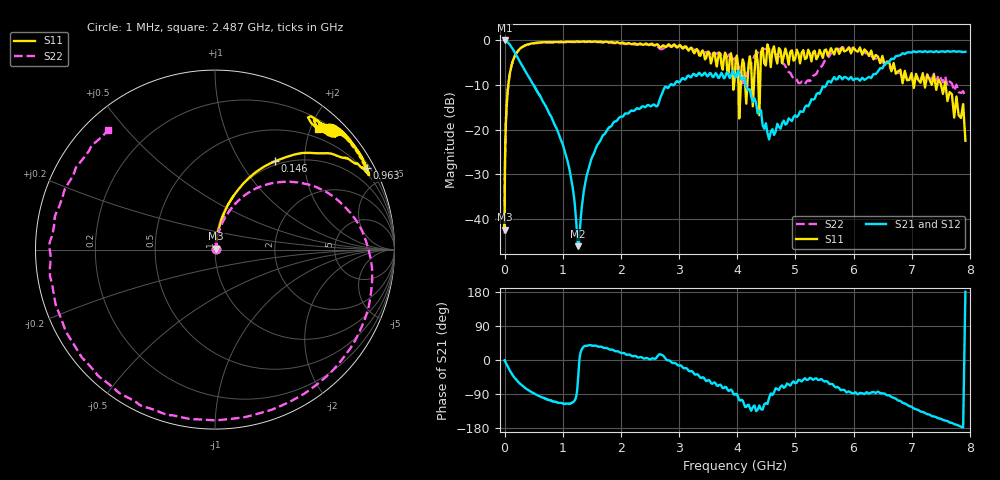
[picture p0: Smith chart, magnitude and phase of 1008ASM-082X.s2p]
!s-Parameter Generated by FASTRON Sdn. Bhd.
!FASTRON P/N : 1008ASM-082X
!Keysight Technologies: E5071C_MY46733604_B.14.02
!Date: Tue Nov 21 11:36:22 2023
!Version  :Rev00  Wed Nov 22 15:52:03 2023
!Data & Calibration Information:
!Freq  S11:SOLT2(ON)  S21:SOLT2(ON)  S12:SOLT2(ON)  S22:SOLT2(ON)
!PortZ  Port1:50+j0  Port2:50+j0
!When reading reference impedance value at option line is always used.
! Remarks : This data is being provided solely for informational purposes.
# Hz S dB R 50
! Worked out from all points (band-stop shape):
!   1599 points, 1 MHz to 7.923 GHz, reference 50 ohm
!   highest |S21| = -0.05 dB at 1.284 MHz (marker M1); lowest = -46.1 dB at 1.264 GHz (marker M2)
!   |S21| within 3 dB of the highest: start of sweep to 188.6 MHz; 6.885 GHz to end of sweep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
!   lowest |S11| = -42.4 dB at 1.31 MHz (marker M3), VSWR 1.02, Z = 50.6 + j0.474 ohm
!   |S11| at or under -10 dB: start of sweep to 64.94 MHz; 4.022 GHz to 4.062 GHz (40.34 MHz wide, 0.998 % of centre); 7.582 GHz to end of sweep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
!   |S22| runs from -43.4 to -0.3 dB; largest |S21 - S12| = 0.013
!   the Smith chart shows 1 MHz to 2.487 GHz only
!   S11 on the Smith chart (normalised r, x): 1 MHz: 1.01, +0.01; 146 MHz: 0.94, +1.43; 963 MHz: 0.35, +3.95; 2.487 GHz: 0.35, +2.11
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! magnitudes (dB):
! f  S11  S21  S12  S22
! 1 MHz  -41.4  -0.1  -0.1  -41.3
! 1.284 MHz  -40.9  0.0  -0.1  -41.9
! 1.31 MHz  -42.4  -0.1  -0.1  -43.4
! 4.479 MHz  -32.1  -0.1  -0.1  -32.1
! 19.95 MHz  -19.6  -0.1  -0.1  -19.5
! 89.01 MHz  -7.6  -1.0  -1.0  -7.7
! 146 MHz  -4.5  -2.1  -2.1  -4.5
! 398.5 MHz  -0.9  -7.8  -7.8  -1.0
! 963 MHz  -0.4  -22.1  -22.1  -0.5
! 1.12 GHz  -0.4  -29.2  -29.2  -0.4
! 1.264 GHz  -0.3  -46.1  -46.1  -0.4
! 1.458 GHz  -0.3  -28.2  -28.2  -0.4
! 1.784 GHz  -0.5  -19.7  -19.7  -0.6
! 2.487 GHz  -1.1  -14.6  -14.6  -1.0
! 3.143 GHz  -2.0  -8.0  -8.0  -1.8
! 3.953 GHz  -9.0  -7.8  -7.9  -4.0
! 4.197 GHz  -5.2  -11.0  -11.0  -6.3
! 4.661 GHz  -3.7  -20.5  -20.4  -3.1
! 5.136 GHz  -2.2  -16.0  -16.0  -9.6
! 6.034 GHz  -2.3  -8.6  -8.6  -2.2
! 7.422 GHz  -11.1  -2.4  -2.4  -9.2
! 7.923 GHz  -22.5  -2.6  -2.6  -12.8
